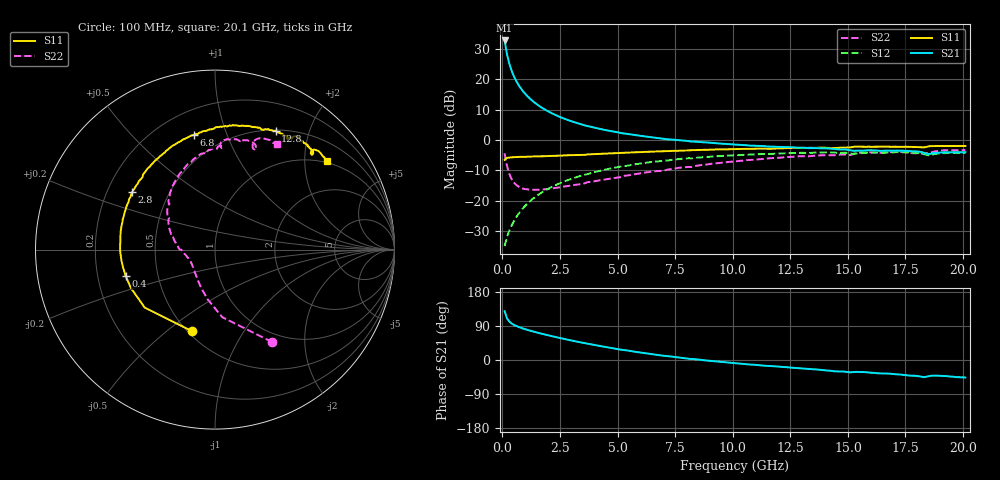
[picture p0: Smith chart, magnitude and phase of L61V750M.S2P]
!  Infineon Technologies AG
! BFR380L3 , PF131585-7, No.6, Th 09.10.01, soldered on pcb-board, measured with PP GSG850
!  Vce=1.75 V,  Ic=50.0 mA
! Common Emitter S-Parameters:  15. November 2001
#  GHz  S  MA  R  50
! f  S11  S21  S12  S22
! GHz  Mag  Ang  Mag  Ang  Mag  Ang  Mag  Ang
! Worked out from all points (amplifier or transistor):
!   201 points, 100 MHz to 20.1 GHz, reference 50 ohm
!   highest |S21| = 32.7 dB at 100 MHz (marker M1)
!   |S21| within 3 dB of that: start of sweep to 167.9 MHz
!   unconditionally stable (mu >= 1): 857.8 MHz to 4.305 GHz
!   at 3.4 GHz: K = 1.02, MAG = 7.7 dB, |S12| = -11.8 dB
!   at 10.1 GHz: K = 0.96, MSG = 1.8 dB, |S12| = -5.0 dB
!   at 20.1 GHz: K = 0.99, MSG = 0.1 dB, |S12| = -4.2 dB
!   S11 on the Smith chart (normalised r, x): 100 MHz: 0.53, -0.61; 400 MHz: 0.32, -0.13; 2.8 GHz: 0.31, +0.29; 6.8 GHz: 0.35, +0.77; 12.8 GHz: 0.51, +1.51; 20.1 GHz: 0.94, +2.57
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0.1  0.4721 -105.7  43.3 129.0  0.01797 58.7  0.6052 -58.3
0.2  0.5077 -140.4  26.03 110.2  0.02524 57.4  0.379 -83.8
0.3  0.5148 -155.3  18.18 101.7  0.03205 61.3  0.2801 -98.4
0.4  0.5191 -163.4  13.88 96.6  0.03897 63.8  0.2296 -109.0
0.5  0.5218 -169.1  11.21 92.8  0.04598 66.1  0.2007 -117.4
0.6  0.5247 -173.2  9.389 89.9  0.05348 67.6  0.1833 -124.1
0.7  0.5266 -176.8  8.087 87.3  0.0608 68.5  0.172 -129.9
0.8  0.5289 -179.8  7.101 85.0  0.0684 69.3  0.1641 -134.7
0.9  0.529 177.6  6.328 83.0  0.0758 69.5  0.1589 -138.8
1.1  0.5317 173.0  5.211 79.3  0.09105 69.5  0.1541 -145.4
1.4  0.5362 167.2  4.126 74.1  0.1136 68.8  0.1517 -152.9
1.8  0.5411 160.3  3.246 67.9  0.1436 67.1  0.1541 -160.2
2.3  0.5495 152.3  2.583 60.8  0.1801 64.2  0.1627 -167.5
2.8  0.5609 145.3  2.163 54.1  0.2157 60.8  0.1738 -173.3
3.5  0.5706 135.8  1.774 45.2  0.2644 55.8  0.1894 -180.0
5.1  0.6084 117.4  1.317 27.7  0.3642 43.7  0.2441 163.6
6.8  0.6499 100.6  1.07 12.8  0.4494 31.4  0.3101 146.2
10.1  0.7085 76.8  0.8404 -8.5  0.5608 9.7  0.4461 119.2
12.8  0.7421 62.9  0.7485 -21.7  0.6141 -6.7  0.5383 98.7
13.5  0.7423 59.4  0.7368 -24.6  0.6188 -10.5  0.5489 94.5
16.8  0.7757 47.6  0.6687 -35.9  0.6226 -25.9  0.6307 75.1
20.1  0.7976 38.4  0.6293 -46.3  0.6164 -39.2  0.6834 59.8
